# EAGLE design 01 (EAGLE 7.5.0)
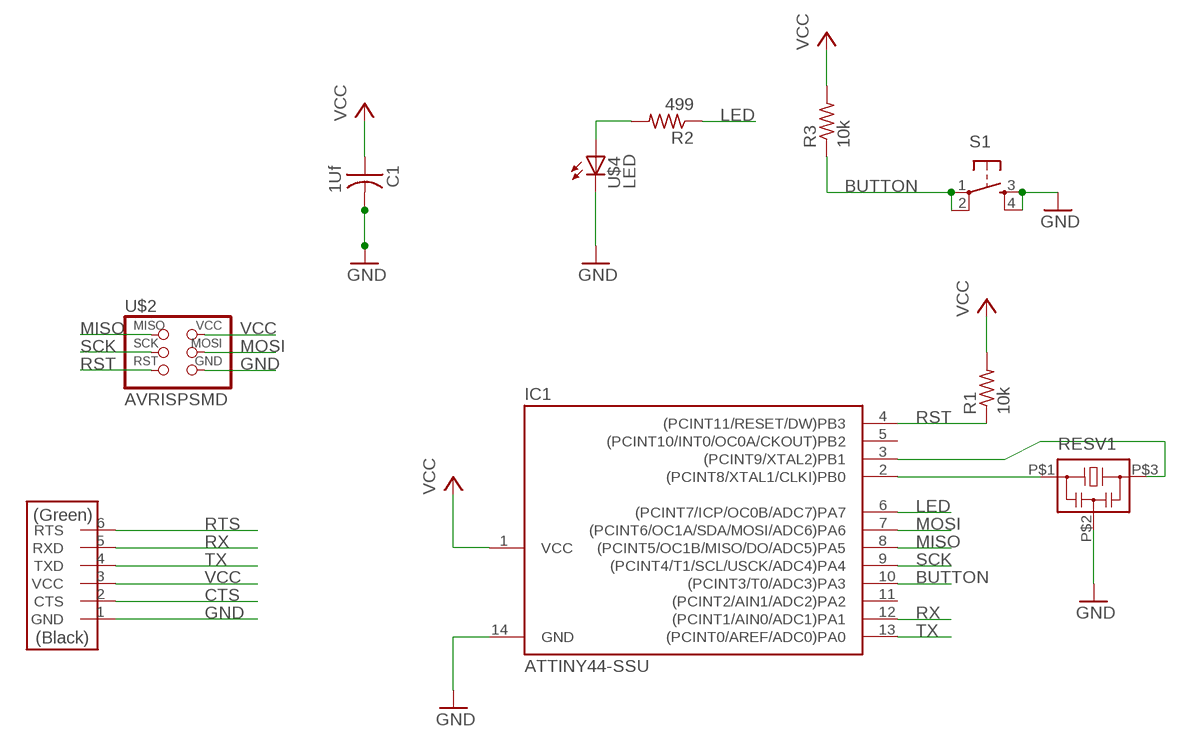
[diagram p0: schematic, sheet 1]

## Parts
C1  1Uf  CAP-US1206FAB  [C1206FAB]
IC1  ATTINY44-SSU  [SOIC14]
R1  10k  RES-US1206FAB  [R1206FAB]
R2  499  RES-US1206FAB  [R1206FAB]
R3  10k  RES-US1206FAB  [R1206FAB]
RESV1  RESONATOR-VOLT  [VOLT]
S1  6MM_SWITCH6MM_SWITCH  [6MM_SWITCH]
U$2  AVRISPSMD  [2X03SMD]
U$3  FTDI-SMD-HEADER  [1X06SMD]
U$4  LED  [LED1206]

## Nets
BUTTON: IC1.10((PCINT3/T0/ADC3)PA3) R3.1 S1.1(P) S1.2(P1)
CTS: U$3.2(CTS)
GND: C1.2 IC1.14(GND) RESV1.P$2 S1.3(S) S1.4(S1) U$2.6(GND) U$3.1(GND) U$4.2(C)
LED: IC1.6((PCINT7/ICP/OC0B/ADC7)PA7) R2.1
MISO: IC1.8((PCINT5/OC1B/MISO/DO/ADC5)PA5) U$2.1(MISO)
MOSI: IC1.7((PCINT6/OC1A/SDA/MOSI/ADC6)PA6) U$2.4(MOSI)
N$1: R2.2 U$4.1(A)
N$3: IC1.3((PCINT9/XTAL2)PB1) RESV1.P$3
N$4: IC1.2((PCINT8/XTAL1/CLKI)PB0) RESV1.P$1
RST: IC1.4((PCINT11/RESET/DW)PB3) R1.1 U$2.5(RST)
RTS: U$3.6(RTS)
RX: IC1.12((PCINT1/AIN0/ADC1)PA1) U$3.5(RXD)
SCK: IC1.9((PCINT4/T1/SCL/USCK/ADC4)PA4) U$2.3(SCK)
TX: IC1.13((PCINT0/AREF/ADC0)PA0) U$3.4(TXD)
VCC: C1.1 IC1.1(VCC) R1.2 R3.2 U$2.2(VCC) U$3.3(VCC)
Unconnected: IC1.5((PCINT10/INT0/OC0A/CKOUT)PB2) IC1.11((PCINT2/AIN1/ADC2)PA2)

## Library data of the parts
C1 = 01_fab:CAP-US
IC1 = 01_fab:ATTINY44
R1-R3 = 01_fab:RES-US: Resistor (US Symbol)
RESV1 = Volt:RESONATOR-VOLT
S1 = 01_fab:6MM_SWITCH: OMRON SWITCH
U$2 = 01_fab:AVRISP
U$3 = 01_fab:FTDI-SMD-HEADER
U$4 = 01_fab:LED: LED

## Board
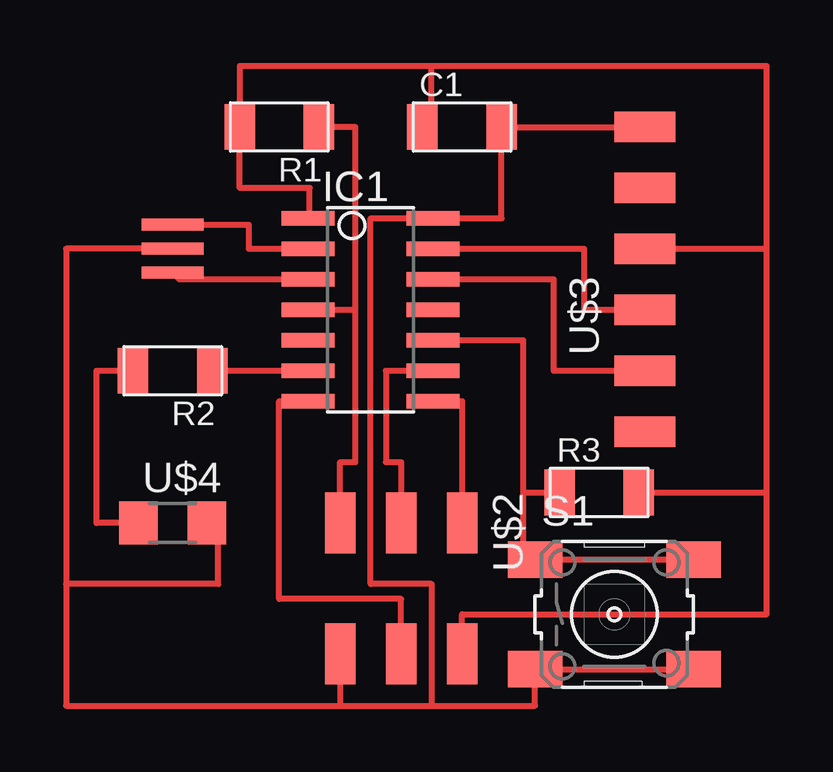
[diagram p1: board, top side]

No outline drawn. Coordinates in mm, seen from the top.
Copper layers (1*16): Top 0.035mm / dielectric 1.5mm / Bottom 0.035mm
Design rules "default *": minimum track width 5mil, minimum drill 24mil, track to track 2.5mil, track to pad 8mil, pad to pad 8mil, via to via 8mil, smd to smd 8mil, copper to edge 40mil, drill to drill 8mil, minimum pad ring 10mil, minimum via ring 8mil, stop-mask expansion 4mil, vias tented up to drill 0mil, thermal gap 10mil

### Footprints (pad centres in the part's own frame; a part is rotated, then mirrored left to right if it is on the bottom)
C1206FAB = smd 1.27 x 1.905: 1 -1.651,0; 2 1.651,0
SOIC14 = smd 0.61 x 2.21: 1 -3.81,-2.603; 2 -2.54,-2.603; 3 -1.27,-2.603; 4 0,-2.603; 5 1.27,-2.603; 6 2.54,-2.603; 7 3.81,-2.603; 8 3.81,2.603; 9 2.54,2.603; 10 1.27,2.603; 11 0,2.603; 12 -1.27,2.603; 13 -2.54,2.603; 14 -3.81,2.603
R1206FAB = smd 1.27 x 1.905: 1 -1.651,0; 2 1.651,0
VOLT = smd 0.5 x 2.6: P$1 -1,0; P$2 0,0; P$3 1,0
6MM_SWITCH = smd 2.286 x 1.524: 1 -3.302,2.286; 2 3.302,2.286; 3 -3.302,-2.286; 4 3.302,-2.286
2X03SMD = smd 2.54 x 1.27: 1 -2.54,2.54; 2 2.92,2.54; 3 -2.54,0; 4 2.92,0; 5 -2.54,-2.54; 6 2.92,-2.54
1X06SMD = smd 2.54 x 1.27: 1 0,6.35; 2 0,3.81; 3 0,1.27; 4 0,-1.27; 5 0,-3.81; 6 0,-6.35
LED1206 = smd 1.6 x 1.803: 1 -1.422,0; 2 1.422,0

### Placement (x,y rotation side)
C1  35.56,33.02 0 top
IC1  31.75,25.4 270 top
R1  27.94,33.02 180 top
R2  23.5,22.86 180 top
R3  41.27,17.78 0 top
RESV1  23.5,27.94 270 top
S1  41.91,12.7 0 top
U$2  33.02,13.97 270 top
U$3  43.18,26.67 0 top
U$4  23.5,16.51 0 top

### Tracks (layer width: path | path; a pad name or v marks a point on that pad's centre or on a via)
BUTTON
  Top 0.254: IC1.10 38.1,24.13 38.1,17.78 | 38.1,17.78 R3.1 | 38.1,17.78 38.1,15.24 38.61,15.24 S1.1 S1.2
GND
  Top 0.254: 19.05,13.97 19.05,27.94 RESV1.P$2 | 19.05,13.97 19.05,8.89 30.48,8.89 | 30.48,8.89 34.29,8.89 | 19.05,13.97 25.4,13.97 25.4,16.51 U$4.2 | 34.29,8.89 34.29,13.97 31.75,13.97 31.75,29.21 IC1.14 37.21,29.21 C1.2 U$3.1 | U$2.6 30.48,8.89 | 34.29,8.89 38.61,8.89 S1.3 S1.4
LED
  Top 0.254: R2.1 IC1.6
MISO
  Top 0.254: IC1.8 35.56,21.59 U$2.1
MOSI
  Top 0.254: U$2.4 33.02,13.34 27.94,13.34 27.94,21.59 IC1.7
N$1
  Top 0.254: U$4.1 20.32,16.51 20.32,22.86 R2.2
  Top 0.406: 21.44,22.86 R2.2
N$3
  Top 0.254: RESV1.P$3 23.77,26.67 IC1.3
  Top 0.406: 29.15,26.59 IC1.3
N$4
  Top 0.254: RESV1.P$1 26.67,28.94 26.67,27.94 IC1.2
RST
  Top 0.254: U$2.5 30.48,19.05 31.11,19.05 31.11,25.4 | 31.11,25.4 31.11,33.02 R1.1 | IC1.4 31.11,25.4
RX
  Top 0.254: IC1.12 39.37,26.67 39.37,22.86 U$3.5
SCK
  Top 0.254: IC1.9 32.38,22.86 32.38,19.05 33.02,19.05 U$2.3
TX
  Top 0.254: IC1.13 40.64,27.94 40.64,25.4 U$3.4
VCC
  Top 0.254: 29.21,29.21 29.21,30.48 26.29,30.48 R1.2 26.29,35.56 34.29,35.56 | C1.1 34.29,33.02 34.29,35.56 | 35.56,11.43 35.56,12.7 48.26,12.7 48.26,17.78 | 48.26,17.78 48.26,27.94 | 48.26,27.94 48.26,35.56 34.29,35.56 | U$3.3 48.26,27.94 | R3.2 48.26,17.78
  Top 0.406: 35.56,11.43 U$2.2 | 29.21,29.21 IC1.1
